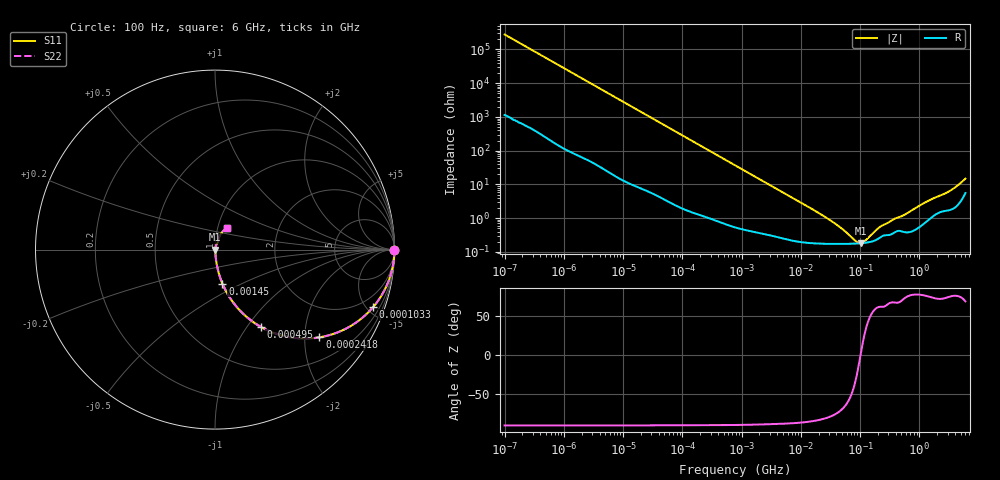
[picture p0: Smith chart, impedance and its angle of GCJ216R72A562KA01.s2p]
!Murata Part Number: GCJ216R72A562KA01
!These Parameters are Measured in Series Mode Connection
!Data Generated on Mar 13, 2026
!  o--ll--o
!Port1  Port2
!  o------o
!Operation Temp=25[degC], DC Bias Voltage=0[V]
!Freq. Start=100[Hz] Stop=6[GHz] 401[Steps]
# Hz S RI R 50
!Freq.(Hz) S11(Real) S11(Imag) S21(Real) S21(Imag) S12(Real) S12(Imag) S22(Real) S22(Imag)
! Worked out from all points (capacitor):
!   401 points, 100 Hz to 6 GHz, reference 50 ohm
!   read as one part in series: C = 5.7 nF near 109 Hz
!   lowest |Z| = 181 mohm at 102 MHz (marker M1)
!   series resonance near 102 MHz, so ESL is about 430 pH
!   S11 on the Smith chart (normalised r, x): 100 Hz: open; 103.3 kHz: 1.04, -5.51; 241.8 kHz: 1.02, -2.36; 495 kHz: 1.01, -1.16; 1.45 MHz: 1.01, -0.40; 6 GHz: 1.11, +0.28
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100  1 -0.000359  1.6e-06 0.000359  1.6e-06 0.000359  1 -0.000359
2008  0.9999 -0.00715  8.38e-05 0.00715  8.38e-05 0.00715  0.9999 -0.00715
12592  0.9978 -0.0445  0.0022 0.0445  0.0022 0.0445  0.9978 -0.0445
40335  0.9793 -0.1392  0.0207 0.1392  0.0207 0.1392  0.9793 -0.1392
103284  0.8819 -0.3193  0.1181 0.3193  0.1181 0.3193  0.8819 -0.3193
154540  0.7709 -0.4164  0.2291 0.4164  0.2291 0.4164  0.7709 -0.4164
241822  0.5815 -0.4887  0.4185 0.4887  0.4185 0.4887  0.5815 -0.4887
495019  0.2537 -0.4291  0.7463 0.4291  0.7463 0.4291  0.2537 -0.4291
774597  0.1245 -0.323  0.8755 0.323  0.8755 0.323  0.1245 -0.323
1449809  0.0417 -0.1898  0.9583 0.1898  0.9583 0.1898  0.0417 -0.1898
3882480  0.00833 -0.0742  0.9917 0.0742  0.9917 0.0742  0.00833 -0.0742
1.555665e7  0.00215 -0.0184  0.9978 0.0184  0.9978 0.0184  0.00215 -0.0184
3.64232e7  0.00178 -0.00706  0.9982 0.00706  0.9982 0.00706  0.00178 -0.00706
8.527865e7  0.00177 -0.00104  0.9982 0.00104  0.9982 0.00104  0.00177 -0.00104
1.020051e8  0.00181 2.6e-06  0.9982 -2.6e-06  0.9982 -2.6e-06  0.00181 2.6e-06
1.220122e8  0.00186 0.00106  0.9981 -0.00106  0.9981 -0.00106  0.00186 0.00106
2.088084e8  0.00256 0.00458  0.9974 -0.00458  0.9974 -0.00458  0.00256 0.00458
3.124326e8  0.00322 0.00704  0.9968 -0.00704  0.9968 -0.00704  0.00322 0.00704
5.59173e8  0.004 0.0118  0.996 -0.0118  0.996 -0.0118  0.004 0.0118
1.369159e9  0.00919 0.0301  0.9908 -0.0301  0.9908 -0.0301  0.00919 0.0301
3.065283e9  0.0198 0.0556  0.9802 -0.0556  0.9802 -0.0556  0.0198 0.0556
6e9  0.0685 0.1219  0.9315 -0.1219  0.9315 -0.1219  0.0685 0.1219
